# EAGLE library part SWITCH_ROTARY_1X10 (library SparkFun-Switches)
10-Position Rotary Switch Single pole, 10 position rotary switch able to select up to 10 different states. SparkFun Products Rotary Switch - 10 Position (COM-13253) Used on SparkFun Decade Resistance Box
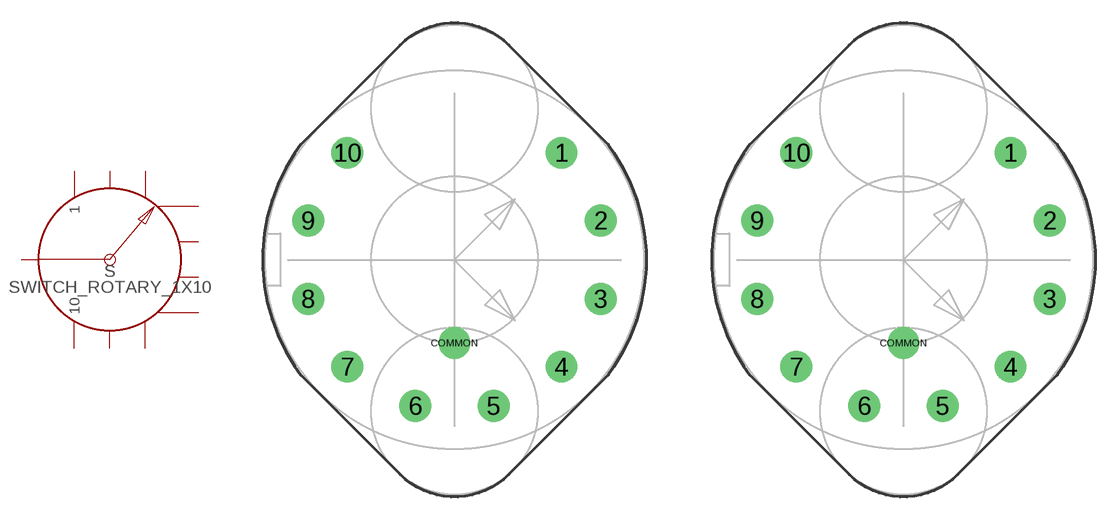
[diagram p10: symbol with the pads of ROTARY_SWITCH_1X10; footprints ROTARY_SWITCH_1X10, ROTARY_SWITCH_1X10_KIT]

Designator prefix S

## SWITCH_ROTARY_1X10-PTH (PROD_ID: SWCH-12120; SF_SKU: COM-13253)  [ROTARY_SWITCH_1X10]
1  1
2  2
3  3
4  4
5  5
6  6
7  7
8  8
9  9
10  10
COMMON  COMMON

## SWITCH_ROTARY_1X10-PTH-KIT (PROD_ID: SWCH-12120; SF_SKU: COM-13253)  [ROTARY_SWITCH_1X10_KIT]
Pads as for ROTARY_SWITCH_1X10

## Footprint ROTARY_SWITCH_1X10 (pad centres in mm)
10-Position Rotary Switch Taiwan Alpha 1 pole, 10 pos rotary switch. Arrows in tDocu denote pointer positions for 45-degree shaft, assuming a knob with a pointer that's opposite the set screw.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
drill 1.4: 1 7.071,7.071; 2 9.659,2.588; 3 9.659,-2.588; 4 7.071,-7.071; 5 2.588,-9.659; 6 -2.588,-9.659; 7 -7.071,-7.071; 8 -9.659,-2.588; 9 -9.659,2.588; 10 -7.071,7.071; COMMON 0,-5.5

## Footprint ROTARY_SWITCH_1X10_KIT (pad centres in mm)
10-Position Rotary Switch - KIT Version Taiwan Alpha 1 pole, 10 pos rotary switch. Arrows in tDocu denote pointer positions for 45-degree shaft, assuming a knob with a pointer that's opposite the set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
drill 1.4: 1 7.071,7.071; 2 9.659,2.588; 3 9.659,-2.588; 4 7.071,-7.071; 5 2.588,-9.659; 6 -2.588,-9.659; 7 -7.071,-7.071; 8 -9.659,-2.588; 9 -9.659,2.588; 10 -7.071,7.071; COMMON 0,-5.5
